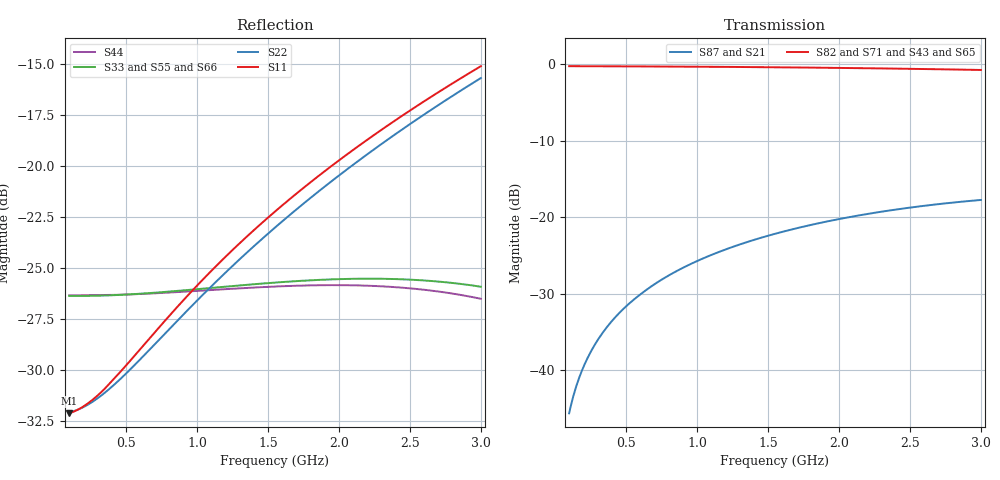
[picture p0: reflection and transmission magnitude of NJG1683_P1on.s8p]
! Created Wed May 22 11:48:09 2013
# hz S ma R 50
! 8 Port Network Data from SP2.SP block
! freq  magS11  angS11  magS12  angS12  magS13  angS13  magS14  angS14
!  magS15  angS15  magS16  angS16  magS17  angS17  magS18  angS18
!  magS21  angS21  magS22  angS22  magS23  angS23  magS24  angS24
!  magS25  angS25  magS26  angS26  magS27  angS27  magS28  angS28
!  magS31  angS31  magS32  angS32  magS33  angS33  magS34  angS34
!  magS35  angS35  magS36  angS36  magS37  angS37  magS38  angS38
!  magS41  angS41  magS42  angS42  magS43  angS43  magS44  angS44
!  magS45  angS45  magS46  angS46  magS47  angS47  magS48  angS48
!  magS51  angS51  magS52  angS52  magS53  angS53  magS54  angS54
!  magS55  angS55  magS56  angS56  magS57  angS57  magS58  angS58
!  magS61  angS61  magS62  angS62  magS63  angS63  magS64  angS64
!  magS65  angS65  magS66  angS66  magS67  angS67  magS68  angS68
!  magS71  angS71  magS72  angS72  magS73  angS73  magS74  angS74
!  magS75  angS75  magS76  angS76  magS77  angS77  magS78  angS78
!  magS81  angS81  magS82  angS82  magS83  angS83  magS84  angS84
!  magS85  angS85  magS86  angS86  magS87  angS87  magS88  angS88
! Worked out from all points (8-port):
!   291 points, 100 MHz to 3 GHz, reference 50 ohm
!   strongest paths, dB at 100 MHz, 820 MHz, 1.55 GHz, 2.28 GHz, 3 GHz:
!     S82: -0.3, -0.3, -0.4, -0.6, -0.8
!     S71: -0.3, -0.3, -0.4, -0.6, -0.8
!     S43: -0.5, -0.5, -0.5, -0.6, -0.6
!     S65: -0.5, -0.5, -0.5, -0.6, -0.6
!     S87: -45.7, -27.4, -22.2, -19.4, -17.8
!     S21: -45.7, -27.5, -22.3, -19.5, -18.0
!   lowest |S11| = -32.1 dB at 100 MHz (marker M1), VSWR 1.05, Z = 52.5 - j0.574 ohm
!   |S11| at or under -10 dB: start of sweep to end of sweep
